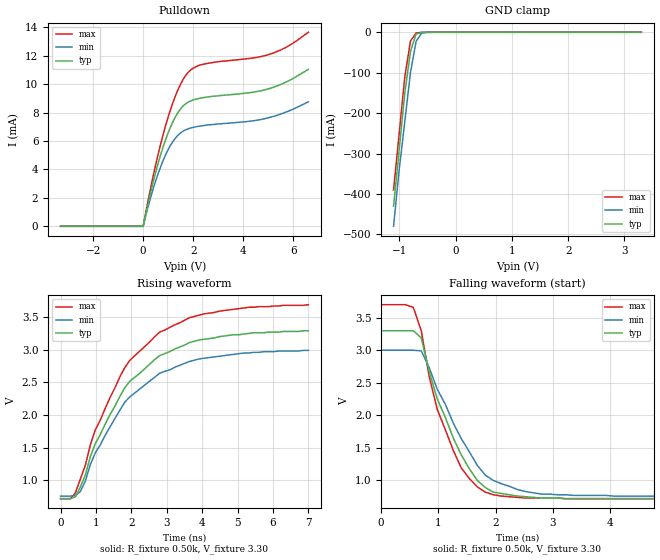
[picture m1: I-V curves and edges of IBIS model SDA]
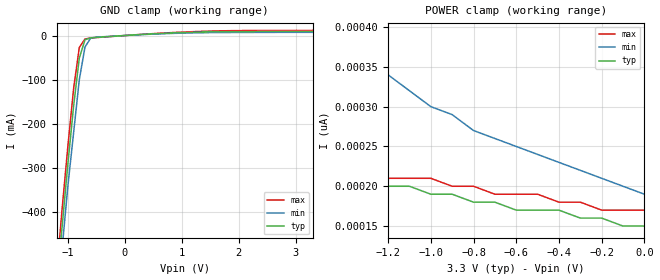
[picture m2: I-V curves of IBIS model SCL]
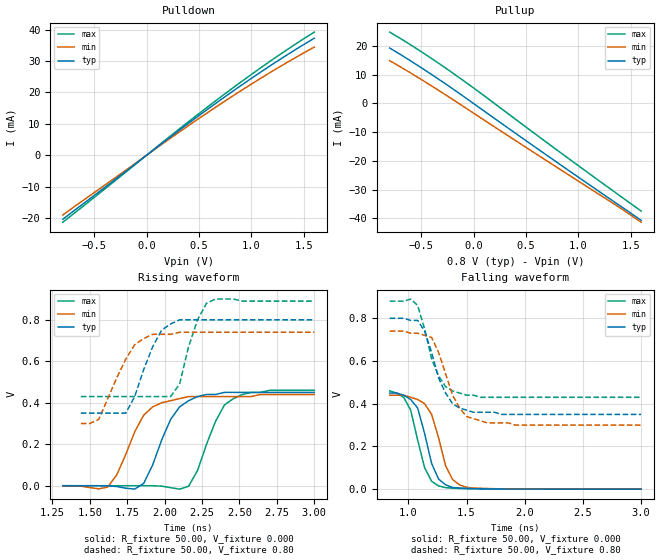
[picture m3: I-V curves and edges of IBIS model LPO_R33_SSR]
| Integrated Devices Technolgy, Inc
[Ibis Ver]   3.2
[File Name]   9lrs4103b.ibs
[File Rev]   1.0
[Date]   10/08/2009
[Source]   Integrated Devices Technolgy, Inc.
[Notes]   Rev 0.0 created by wm
[Disclaimer] Integrated Device Technology, Inc. ("IDT") hereby grants the
   user of this IBIS model a non-exclusive, nontransferable
   license to use this IBIS model under the following terms. The
   user is granted this license only to use the IBIS model and is
   not granted rights to sell, copy (except as needed to run the
   IBIS model), rent, lease or sub-license the IBIS model in
   whole or in part, or in modified form to anyone. The User may
   modify the IBIS model to suit its specific applications, but
   rights to derivative works and such modifications shall belong
   to IDT. This IBIS model is provided on an AS IS" basis and IDT
   makes absolutely no warranty with respect to the information
   contained herein. IDT DISCLAIMS AND CUSTOMER WAIVES ALL
   WARRANTIES, EXPRESS AND IMPLIED, INCLUDING WARRANTIES OF
   MERCHANTABILITY AND FITNESS FOR A PARTICULAR PURPOSE. THE
   ENTIRE RISK AS TO QUALITY AND PERFORMANCE IS WITH THE USER
   ACCORDINGLY, IN NO EVENT SHALL IDT BE LIABLE FOR ANY DIRECT OR
   INDIRECT DAMAGES, WHETHER IN CONTRACT OR TORT, INCLUDING ANY
   LOST PROFITS OR OTHER INCIDENTAL, CONSEQUENTIAL, EXEMPLARY, OR
   PUNITIVE DAMAGES ARISING OUT OF THE USE OR APPLICATION OF THE
   IBIS model. Further, IDT reserves the right to make changes
   without notice to any product herein to improve reliability,
   function, or design. IDT does not convey any license under
   patent rights or any other intellectual property rights,
   including those of third parties. IDT is not obligated to
   provide maintenance or support for the licensed IBIS model.
[Copyright]   Copyright 2006, Integrated Devices Technolgy, Inc. all rights
   reserved
|   COMPONENT: 9LRS4103
[Component]   IDT9LRS4103
[Manufacturer]   Integrated Device Technology, Inc.
[Package]
| variable   typ   min   max
R_pkg   81.1m   62.2m   100.0m
L_pkg   6.7nH   4.9nH   8.5nH
C_pkg   0.53pF   0.21pF   0.85pF
[Pin]  signal_name   model_name   R_pin   L_pin   C_pin
1   X1   XT1
2   X2   XT1
3   SCLK   SCL
4   SDATA   SDA
5   VDD   POWER
6   DOT96T   LPO_R33_SSR
7   DOT96C   LPO_R33_SSR
8   GND   GND
9   GND   GND
10   SSC_DISPT   LPO_R33_SSR
11   SSC_DISPC   LPO_R33_SSR
12   VDD   POWER
13   VDD   POWER
14   SRC1_SATA_NST   LPO_R33_SSR
15   SRC1_SATA_NSC   LPO_R33_SSR
16   GND   GND
17   GND   GND
18   SRC2T   LPO_R33_SSR
19   SRC2C   LPO_R33_SSR
20   VDD   POWER
21   SEL_120MB   LPOEM_2X3SR_IN
22   GND   GND
23   CPU0T   LPO_R33_SSR
24   CPU0C   LPO_R33_SSR
25   VDD   POWER
26   VTTPWG_PDB   LPOEM_2X3SR_IN
27   VDD   POWER
28   FSLC_REF   IO_LPOEM_2X3X_SR_PD
29   GND   GND
30   VDD   POWER
31   SEL_SATA_NSB   LPOEM_2X3SR_IN
32   GND   GND
[Diff Pin]   inv_pin   vdiff   tdelay_typ   tdelay_min   tdelay_max
6   7   NA   NA
10   11   NA   NA
14   15   NA   NA
18   25   NA   NA
19   29   NA   NA
23   24   NA   NA
| Models and submodels in the file (6): SDA (I/O_open_drain), SCL (Input), LPO_R33_SSR (Output), XT1 (Input), LPOEM_2X3SR_IN (Input), IO_LPOEM_2X3X_SR_PD (I/O)
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|   Model SDA
[Model]   SDA
Model_type   I/O_open_drain
Polarity   Inverting
Enable   Active-High
Vinl =   0.80V
Vinh =   2.00V
Vmeas =   1.50V
Cref =   5.00pF
Rref =  0.000
Vref =   1.50V
C_comp   3.40pF   2.85pF   3.95pF
[Temperature Range]   27.00   70.00   0.000
[Voltage Range]   3.30V   3.00V   3.70V
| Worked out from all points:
|   slope of the pulldown table from 0 to 0.495 V, typ, clamps not added: 131 ohm
|   GND clamp passes 1 mA (typ) near -0.62 V on its own axis
|   rising waveform, R_fixture 0.50k, V_fixture 3.30: 20-80 % time 1.74ns typ, 1.76ns min, 1.73ns max; typ from 0.72 V to 3.29 V
|   falling waveform, R_fixture 0.50k, V_fixture 3.30: 20-80 % time 693ps typ, 785ps min, 596ps max; typ from 3.3 V to 0.72 V
[Pulldown]
| voltage   I(typ)   I(min)   I(max)
-3.3V     0A         0A         0A
0V        0A         0A         0A
500mV     3.8mA      3.19mA     4.32mA
900mV     6.11mA     5.04mA     7.1mA
1.2V      7.4mA      5.99mA     8.75mA
1.4V      8.03mA     6.42mA     9.64mA
1.8V      8.74mA     6.86mA     10.83mA
2.1V      8.94mA     7mA        11.22mA
2.5V      9.08mA     7.11mA     11.44mA
5.1V      9.72mA     7.68mA     12.13mA
5.7V      10.14mA    8.03mA     12.58mA
6.6V      11.04mA    8.76mA     13.65mA
[GND_clamp]
| voltage   I(typ)   I(min)   I(max)
  |-3.30   -3.78A   -3.64A   -3.87A
  |-3.20   -3.62A   -3.50A   -3.71A
  |-3.10   -3.47A   -3.35A   -3.55A
  |-3.00   -3.31A   -3.21A   -3.39A
  |-2.90   -3.16A   -3.06A   -3.23A
  |-2.80   -3.01A   -2.91A   -3.07A
  |-2.70   -2.85A   -2.77A   -2.91A
  |-2.60   -2.70A   -2.62A   -2.75A
  |-2.50   -2.54A   -2.48A   -2.59A
  |-2.40   -2.39A   -2.33A   -2.43A
  |-2.30   -2.24A   -2.19A   -2.27A
  |-2.20   -2.08A   -2.04A   -2.11A
  |-2.10   -1.93A   -1.90A   -1.95A
  |-2.00   -1.78A   -1.75A   -1.79A
  |-1.90   -1.62A   -1.61A   -1.63A
  |-1.80   -1.47A   -1.46A   -1.47A
  |-1.70   -1.32A   -1.32A   -1.32A
  |-1.60   -1.17A   -1.18A   -1.16A
  |-1.50   -1.02A   -1.03A   -1.00A
  |-1.40   -0.87A   -0.89A   -0.85A
  |-1.30   -0.72A   -0.75A   -0.69A
  |-1.20   -0.57A   -0.61A   -0.54A
-1.1V     -430mA     -480mA     -390mA
-1V       -290mA     -340mA     -250mA
-900mV    -150mA     -220mA     -110mA
-800mV    -47.73mA   -100mA     -21.74mA
-700mV    -4.4mA     -22.46mA   -1.7mA
-600mV    -390uA     -1.82mA    -190uA
-400mV    -1.59uA    -9.25uA    -420nA
3.3V      150pA      220pA      150pA
[Ramp]
| variable   typ   min   max
dV/dt_r   0.27/0.19n   0.21/0.19n   0.35/0.18n
dV/dt_f   0.27/0.21n   0.21/0.22n   0.35/0.20n
[Rising Waveform]
R_fixture = 0.50k
V_fixture = 3.30
V_fixture_min = 3.00
V_fixture_max = 3.70
| time   V(typ)   V(min)   V(max)
0s        720mV      760mV      720mV
280ps     720mV      760mV      720mV
420ps     750mV      770mV      810mV
560ps     900mV      830mV      1.02V
700ps     1.08V      990mV      1.23V
980ps     1.56V      1.42V      1.77V
1.82ns    2.42V      2.2V       2.73V
2.8ns     2.91V      2.64V      3.27V
4.06ns    3.16V      2.87V      3.55V
7ns       3.29V      2.99V      3.69V
[Falling Waveform]
R_fixture = 0.50k
V_fixture = 3.30
V_fixture_min = 3.00
V_fixture_max = 3.70
| time   V(typ)   V(min)   V(max)
0s        3.3V       3V         3.7V
560ps     3.3V       3V         3.66V
700ps     3.19V      2.99V      3.3V
840ps     2.67V      2.73V      2.59V
980ps     2.25V      2.4V       2.09V
1.4ns     1.39V      1.64V      1.19V
1.68ns    1V         1.23V      900mV
1.82ns    890mV      1.08V      820mV
2.8ns     730mV      790mV      730mV
7ns       720mV      760mV      720mV
|   Model SCL
[Model]   SCL
Model_type   Input
Polarity   Inverting
Enable   Active-High
Vinl =   0.80V
Vinh =   2.00V
C_comp   3.40pF   2.85pF   3.95pF
[Temperature Range]   27.00   70.00   0.000
[Voltage Range]   3.30V   3.00V   3.70V
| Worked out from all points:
|   GND clamp passes 1 mA (typ) near -0.12 V on its own axis
[GND_clamp]
| voltage   I(typ)   I(min)   I(max)
-3.3V     -3.78A     -3.64A     -3.87A
-1.2V     -570mA     -610mA     -540mA
-1.1V     -430mA     -480mA     -390mA
-1V       -290mA     -340mA     -250mA
-900mV    -160mA     -220mA     -120mA
-800mV    -50.98mA   -100mA     -26.96mA
-700mV    -9.68mA    -25.77mA   -7.88mA
-600mV    -5.33mA    -5.93mA    -5.67mA
-400mV    -3.36mA    -2.92mA    -3.72mA
600mV     4.44mA     3.71mA     5.07mA
1.4V      8.03mA     6.42mA     9.64mA
3.3V      9.23mA     7.24mA     11.63mA
[POWER_clamp]
| voltage   I(typ)   I(min)   I(max)
-3.3V     350pA      1.67nA     310pA
-2.6V     280pA      890pA      270pA
-2.5V     280pA      820pA      270pA
-2.4V     270pA      750pA      260pA
-2.2V     250pA      640pA      260pA
-1.7V     230pA      450pA      230pA
-1.5V     220pA      400pA      230pA
-1.4V     210pA      380pA      220pA
-1V       190pA      300pA      210pA
-800mV    180pA      270pA      200pA
-200mV    160pA      210pA      170pA
0V        150pA      190pA      170pA
|   Model LPO_R33_SSR
[Model]   LPO_R33_SSR
Model_type   Output
Polarity   Inverting
Vmeas =   0.40V
Cref =   2.00pF
Rref =  0.000
Vref =   0.40V
C_comp   3.40pF   2.85pF   3.95pF
[Temperature Range]   27.00   70.00   0.000
[Voltage Range]   0.80V   0.66V   1.00V
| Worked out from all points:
|   slope of the pulldown table from 0 to 0.12 V, typ, clamps not added: 38.7 ohm
|   slope of the pullup table from 0 to 0.12 V, typ, clamps not added: 38.5 ohm
|   rising waveform, R_fixture 50.00, V_fixture 0.000: 20-80 % time 167ps typ, 176ps min, 155ps max; typ from 0 V to 0.45 V
|   rising waveform, R_fixture 50.00, V_fixture 0.80: 20-80 % time 145ps typ, 175ps min, 108ps max; typ from 0.35 V to 0.8 V
|   falling waveform, R_fixture 50.00, V_fixture 0.000: 20-80 % time 135ps typ, 143ps min, 127ps max; typ from 0.45 V to 0 V
|   falling waveform, R_fixture 50.00, V_fixture 0.80: 20-80 % time 174ps typ, 182ps min, 154ps max; typ from 0.8 V to 0.35 V
[Pulldown]
| voltage   I(typ)   I(min)   I(max)
-800mV    -20.43mA   -19.07mA   -21.37mA
200mV     5.15mA     4.77mA     5.4mA
700mV     17.5mA     16.21mA    18.38mA
1.2V      28.96mA    26.79mA    30.45mA
1.6V      37.29mA    34.46mA    39.24mA
[Pullup]
| voltage   I(typ)   I(min)   I(max)
-800mV    19.3mA     14.89mA    24.84mA
-500mV    12.47mA    8.38mA     18.05mA
-100mV    2.59mA     -960uA     8.05mA
900mV     -23.1mA    -24.66mA   -18.97mA
1.4V      -35.64mA   -36.35mA   -32.2mA
1.6V      -40.66mA   -41.3mA    -37.43mA
[Ramp]
| variable   typ   min   max
dV/dt_r   0.27/0.16n   0.26/0.17n   0.28/0.15n
dV/dt_f   0.27/0.16n   0.26/0.17n   0.27/0.14n
R_load = 50.00
[Rising Waveform]
R_fixture = 50.00
V_fixture = 0.000
V_fixture_min = 0.000
V_fixture_max = 0.000
| time   V(typ)   V(min)   V(max)
|  0.000S   0.000V   0.000V   0.000V
|  60.00pS   0.000V   0.000V   0.000V
|   0.12nS   0.000V   0.000V   0.000V
|   0.18nS   0.000V   0.000V   0.000V
|   0.24nS   0.000V   0.000V   0.000V
|   0.30nS   0.000V   0.000V   0.000V
|   0.36nS   0.000V   0.000V   0.000V
|   0.42nS   0.000V   0.000V   0.000V
1.32ns    0V         1.74uV     0V
1.62ns    -380uV     -6.38mV    0V
1.68ns    -3.76mV    52.01mV    0V
1.8ns     -16.39mV   260mV      0V
1.86ns    11mV       340mV      590nV
2.04ns    320mV      410mV      -9.42mV
2.16ns    410mV      430mV      -2.75mV
2.4ns     450mV      430mV      390mV
2.58ns    450mV      430mV      450mV
3ns       450mV      440mV      460mV
[Rising Waveform]
R_fixture = 50.00
V_fixture = 0.80
V_fixture_min = 0.66
V_fixture_max = 1.00
| time   V(typ)   V(min)   V(max)
|  0.000S   0.35V   0.30V   0.43V
|  60.00pS   0.35V   0.30V   0.43V
|   0.12nS   0.35V   0.30V   0.43V
|   0.18nS   0.35V   0.30V   0.43V
|   0.24nS   0.35V   0.30V   0.43V
|   0.30nS   0.35V   0.30V   0.43V
|   0.36nS   0.35V   0.30V   0.43V
|   0.42nS   0.35V   0.30V   0.43V
|   0.48nS   0.35V   0.30V   0.43V
|   0.54nS   0.35V   0.30V   0.43V
|   0.60nS   0.35V   0.30V   0.43V
|   0.66nS   0.35V   0.30V   0.43V
|   0.72nS   0.35V   0.30V   0.43V
|   0.78nS   0.35V   0.30V   0.43V
|   0.84nS   0.35V   0.30V   0.43V
|   0.90nS   0.35V   0.30V   0.43V
|   0.96nS   0.35V   0.30V   0.43V
|   1.02nS   0.35V   0.30V   0.43V
|   1.08nS   0.35V   0.30V   0.43V
|   1.14nS   0.35V   0.30V   0.43V
|   1.20nS   0.35V   0.30V   0.43V
|   1.26nS   0.35V   0.30V   0.43V
|   1.32nS   0.35V   0.30V   0.43V
|   1.38nS   0.35V   0.30V   0.43V
1.44ns    350mV      300mV      430mV
1.56ns    350mV      320mV      430mV
1.74ns    350mV      610mV      430mV
1.8ns     430mV      680mV      430mV
1.92ns    670mV      730mV      430mV
2.04ns    780mV      730mV      430mV
2.1ns     800mV      740mV      490mV
2.22ns    800mV      740mV      800mV
2.28ns    800mV      740mV      880mV
3ns       800mV      740mV      890mV
[Falling Waveform]
R_fixture = 50.00
V_fixture = 0.000
V_fixture_min = 0.000
V_fixture_max = 0.000
| time   V(typ)   V(min)   V(max)
|  0.000S   0.45V   0.44V   0.46V
|  60.00pS   0.45V   0.44V   0.46V
|   0.12nS   0.45V   0.44V   0.46V
|   0.18nS   0.45V   0.44V   0.46V
|   0.24nS   0.45V   0.44V   0.46V
|   0.30nS   0.45V   0.44V   0.46V
|   0.36nS   0.45V   0.44V   0.46V
|   0.42nS   0.45V   0.44V   0.46V
|   0.48nS   0.45V   0.44V   0.46V
|   0.54nS   0.45V   0.44V   0.46V
|   0.60nS   0.45V   0.44V   0.46V
|   0.66nS   0.45V   0.44V   0.46V
|   0.72nS   0.45V   0.44V   0.46V
|   0.78nS   0.45V   0.44V   0.46V
840ps     450mV      440mV      460mV
960ps     440mV      440mV      430mV
1.02ns    420mV      430mV      370mV
1.08ns    380mV      420mV      230mV
1.14ns    260mV      400mV      100mV
1.2ns     120mV      350mV      36.72mV
1.26ns    47.25mV    240mV      15.16mV
1.38ns    7.82mV     45.18mV    4.66mV
1.5ns     3.77mV     8.36mV     2.34mV
3ns       0V         820nV      0V
[Falling Waveform]
R_fixture = 50.00
V_fixture = 0.80
V_fixture_min = 0.66
V_fixture_max = 1.00
| time   V(typ)   V(min)   V(max)
|  0.000S   0.80V   0.74V   0.88V
|  60.00pS   0.80V   0.74V   0.88V
|   0.12nS   0.80V   0.74V   0.88V
|   0.18nS   0.80V   0.74V   0.88V
|   0.24nS   0.80V   0.74V   0.88V
|   0.30nS   0.80V   0.74V   0.88V
|   0.36nS   0.80V   0.74V   0.88V
|   0.42nS   0.80V   0.74V   0.88V
|   0.48nS   0.80V   0.74V   0.88V
|   0.54nS   0.80V   0.74V   0.88V
|   0.60nS   0.80V   0.74V   0.88V
|   0.66nS   0.80V   0.74V   0.88V
|   0.72nS   0.80V   0.74V   0.88V
|   0.78nS   0.80V   0.74V   0.88V
840ps     800mV      740mV      880mV
1.02ns    790mV      730mV      890mV
1.08ns    790mV      730mV      860mV
1.14ns    740mV      720mV      750mV
1.2ns     640mV      710mV      610mV
1.26ns    520mV      640mV      530mV
1.38ns    400mV      440mV      460mV
1.5ns     370mV      340mV      440mV
1.68ns    360mV      310mV      430mV
3ns       350mV      300mV      430mV
